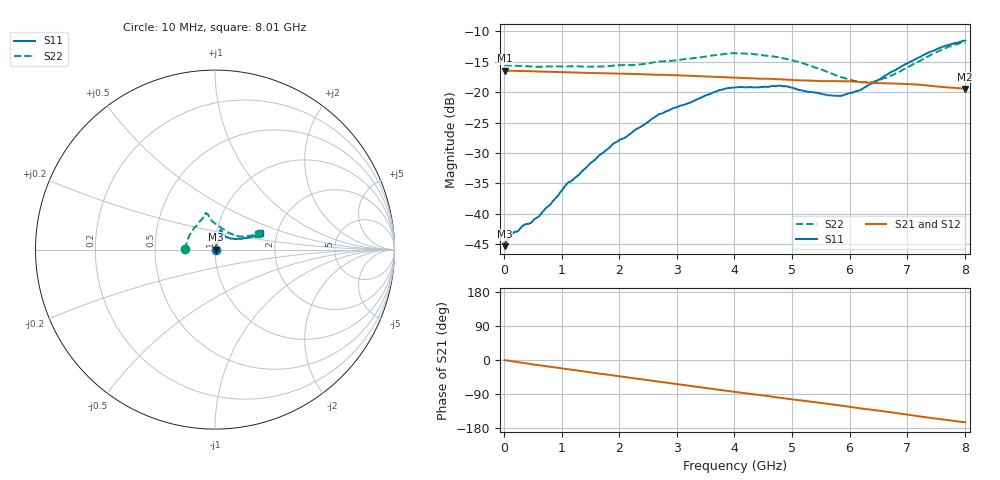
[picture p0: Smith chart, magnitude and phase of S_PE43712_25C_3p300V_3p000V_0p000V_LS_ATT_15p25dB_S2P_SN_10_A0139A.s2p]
! DEVICE ID: PE43712
! File Path: z:\PE43713\PE43713_CHAR_NOM_04292014\AMB\3p300\LS_ATT_15p25dB\PE43713_AMB_3p300V_3p000V_0p000V_LS_ATT_15p25dB_S2P_SN_10_A0139A.s2p
! Serial: 10
! Lot: A0139A
! Temp: 25C
! VDD: 3.300
! VSS: 0.000
! Control_Hi: 3.000
! Control_Lo: 0.000
! Attenuation Step: 15.25dB
! Port 1: RF1
! Port 2: RF2
! ThroughPath:1-2
! IDD: 0.0001475418
! ISS: -1.046e-007
#  Hz  S  RI  R  50
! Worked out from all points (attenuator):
!   801 points, 10 MHz to 8.01 GHz, reference 50 ohm
!   highest |S21| = -16.46 dB at 10 MHz (marker M1); lowest = -19.5 dB at 8 GHz (marker M2)
!   lowest |S11| = -45.3 dB at 10 MHz (marker M3), VSWR 1.01, Z = 50.5 + j0.0444 ohm
!   |S11| at or under -10 dB: start of sweep to end of sweep
!   |S22| runs from -18.4 to -11.8 dB; largest |S21 - S12| = 0.00053
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1e7  0.00541 0.000439  0.1503 -0.000753  0.1504 -0.000734  -0.167 0.00114
1.6e8  0.00651 0.00237  0.1495 -0.00994  0.1496 -0.00994  -0.1647 0.0115
6.1e8  0.00606 0.00739  0.1435 -0.0355  0.1436 -0.0356  -0.1575 0.0376
9.2e8  0.00512 0.0128  0.137 -0.0515  0.1371 -0.0515  -0.153 0.0555
1.09e9  0.00512 0.0169  0.1327 -0.0595  0.1328 -0.0596  -0.1488 0.0661
1.35e9  0.00609 0.0215  0.1257 -0.0712  0.1257 -0.0712  -0.142 0.0794
1.9e9  0.0117 0.036  0.1077 -0.0932  0.1077 -0.0932  -0.122 0.1117
2.33e9  0.0184 0.0473  0.0908 -0.1077  0.0908 -0.1077  -0.1033 0.1328
2.68e9  0.0256 0.0603  0.0757 -0.1164  0.0757 -0.1164  -0.0861 0.1567
3.72e9  0.032 0.0981  0.0269 -0.1306  0.0268 -0.1306  -0.0554 0.1954
4.01e9  0.032 0.1048  0.0133 -0.1311  0.0133 -0.1311  -0.053 0.2024
4.79e9  0.0326 0.1084  -0.0214 -0.126  -0.0214 -0.1261  -0.0361 0.1892
5.35e9  0.0437 0.0898  -0.0435 -0.1164  -0.0434 -0.1164  -0.0186 0.1619
5.87e9  0.0637 0.0687  -0.063 -0.1059  -0.0629 -0.1059  0.0202 0.1309
6.16e9  0.0816 0.0628  -0.0732 -0.0964  -0.073 -0.0966  0.0491 0.1111
6.29e9  0.0932 0.0608  -0.0765 -0.0925  -0.0763 -0.0925  0.0641 0.1017
6.41e9  0.1024 0.0603  -0.0795 -0.0889  -0.0794 -0.0889  0.077 0.0934
6.68e9  0.1298 0.0598  -0.0867 -0.0801  -0.0865 -0.0801  0.1083 0.0797
7.37e9  0.1995 0.0705  -0.1002 -0.0527  -0.1001 -0.0527  0.1831 0.0751
7.71e9  0.2312 0.0789  -0.1022 -0.0396  -0.1021 -0.0397  0.2209 0.0822
8e9  0.2501 0.089  -0.1025 -0.0291  -0.1024 -0.0292  0.2405 0.0865
8.01e9  0.2507 0.0897  -0.1025 -0.0289  -0.1024 -0.029  0.241 0.0864
